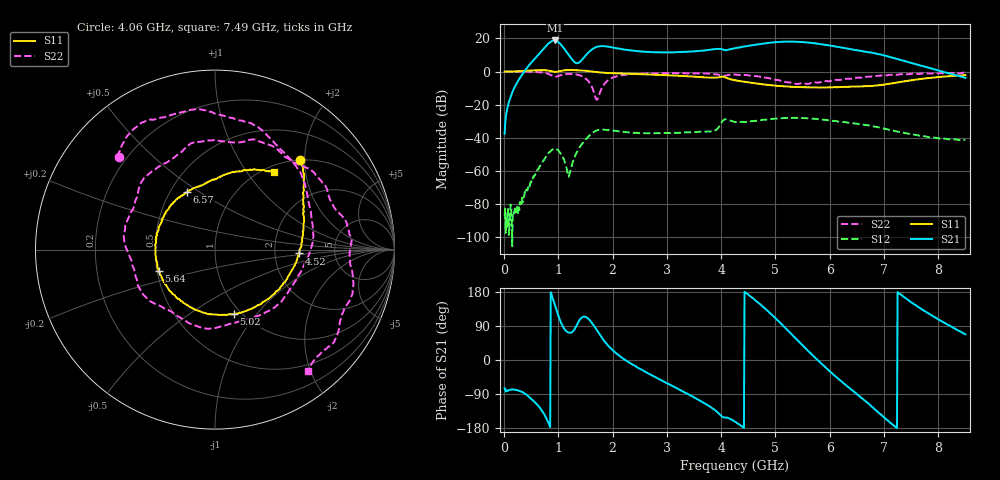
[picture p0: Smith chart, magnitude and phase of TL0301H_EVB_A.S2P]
!Agilent Technologies,E5071C,MY46523237,B.13.01
!Date: Tue Jan 11 12:29:02 2022
!Data & Calibration Information:
!Freq	S11:SOLT2(ON)	S21:SOLT2(ON)	S12:SOLT2(ON)	S22:SOLT2(ON)
!PortZ  Port1:50+j0  Port2:50+j0
!Above PortZ is port z conversion or system Z0 setting when saving the data.
!When reading, reference impedance value at option line is always used.
# Hz S dB R 50
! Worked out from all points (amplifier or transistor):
!   850 points, 10 MHz to 8.5 GHz, reference 50 ohm
!   highest |S21| = 18.8 dB at 940 MHz (marker M1)
!   |S21| within 3 dB of that: 4.548 GHz to 5.989 GHz (1.441 GHz wide, 27.3 % of centre)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
!   unconditionally stable (mu >= 1): 18.31 MHz to 25.47 MHz; 65.68 MHz to 72.83 MHz; 2.169 GHz to end of sweep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
!   at 1.42 GHz: K = -2.45, MSG = 25.5 dB, |S12| = -44.4 dB
!   at 4.26 GHz: K = 1.16, MAG = 19.9 dB, |S12| = -30.4 dB
!   at 8.5 GHz: K = 5.53, MAG = 8.3 dB, |S12| = -41.2 dB
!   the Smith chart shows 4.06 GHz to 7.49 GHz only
!   S11 on the Smith chart (normalised r, x): 4.06 GHz: 1.01, +1.90; 4.52 GHz: 2.74, -0.15; 5.02 GHz: 0.92, -0.77; 5.64 GHz: 0.51, -0.14; 6.57 GHz: 0.61, +0.45; 7.49 GHz: 1.10, +1.35
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1e7  -0.07 -1.0  -37.60 -74.8  -87.03 132.0  0.07 -0.6
5e8  0.67 -43.6  5.35 -102.1  -66.84 -175.9  -0.14 -38.6
7.4e8  0.84 -68.2  14.22 -142.9  -53.05 155.5  -0.77 -60.9
8.6e8  0.33 -81.0  18.00 179.1  -47.98 119.0  -2.12 -71.1
9.4e8  -0.12 -85.4  18.79 143.6  -46.60 85.6  -3.09 -70.4
1.12e9  0.84 -99.2  13.27 80.3  -54.94 34.6  -1.59 -78.4
1.43e9  0.63 -130.6  6.93 111.7  -44.05 114.0  -2.69 -127.1
1.75e9  -0.42 -156.8  15.27 69.8  -35.15 38.6  -14.21 27.9
2.03e9  -0.99 -173.8  14.34 22.3  -35.73 -15.3  -3.31 -63.3
2.84e9  -2.00 136.6  11.64 -49.4  -37.21 -83.8  -1.06 -142.1
4.06e9  -3.27 46.4  13.00 -151.8  -28.95 -149.2  -2.60 135.9
4.26e9  -5.25 25.3  14.15 -163.3  -30.43 172.1  -1.79 118.1
4.52e9  -6.61 -2.6  15.65 169.9  -30.22 148.7  -2.39 90.5
5.02e9  -8.54 -73.7  17.81 107.9  -28.33 95.4  -5.03 13.4
5.3e9  -9.22 -116.2  18.09 67.9  -27.96 58.8  -6.83 -48.0
5.64e9  -9.53 -159.4  17.38 18.7  -28.40 14.0  -7.08 -135.9
5.67e9  -9.48 -162.5  17.31 14.8  -28.44 10.4  -6.68 -141.9
6.11e9  -9.48 155.4  15.07 -43.3  -29.90 -44.8  -5.03 131.7
6.57e9  -8.93 115.7  12.53 -98.3  -31.84 -104.1  -3.70 56.3
7.09e9  -7.39 81.0  9.00 -162.6  -35.13 -174.1  -2.05 -12.8
7.49e9  -5.32 52.9  5.30 153.3  -37.76 137.2  -1.40 -52.7
8.5e9  -2.17 -9.4  -3.76 67.6  -41.17 32.0  -0.69 -124.2
